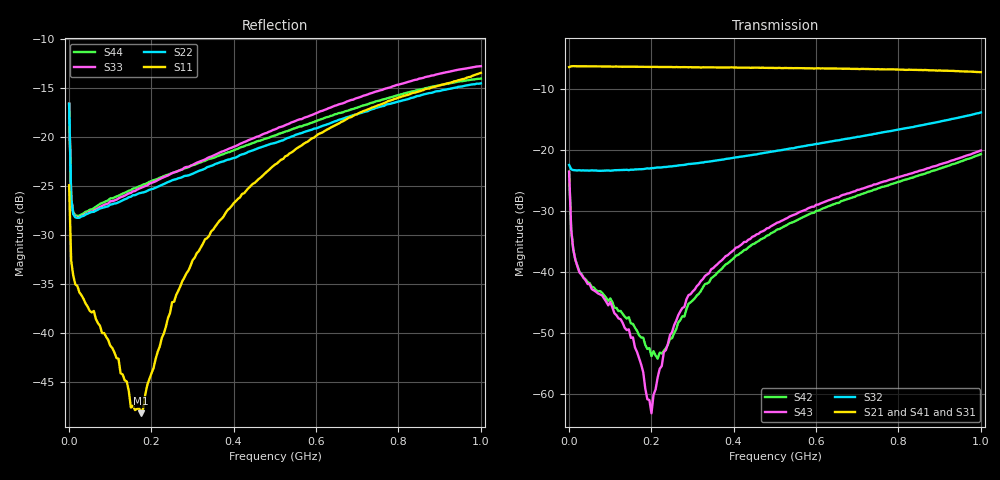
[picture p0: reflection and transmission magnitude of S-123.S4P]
!Agilent Technologies,E5071B,MY42300999,A.09.10
!Date: Thu Apr 13 17:00:39 2023
!Data & Calibration Information:
!Freq	S11:SOLT4(ON)	S12:SOLT4(ON)	S13:SOLT4(ON)	S14:SOLT4(ON)
!	S21:SOLT4(ON)	S22:SOLT4(ON)	S23:SOLT4(ON)	S24:SOLT4(ON)
!	S31:SOLT4(ON)	S32:SOLT4(ON)	S33:SOLT4(ON)	S34:SOLT4(ON)
!	S41:SOLT4(ON)	S42:SOLT4(ON)	S43:SOLT4(ON)	S44:SOLT4(ON)
# Hz S dB R 50
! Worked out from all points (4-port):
!   201 points, 1 MHz to 1 GHz, reference 50 ohm
!   strongest paths, dB at 1 MHz, 250.8 MHz, 500.5 MHz, 750.2 MHz, 1 GHz:
!     S21: -6.4, -6.4, -6.5, -6.7, -7.2
!     S41: -6.4, -6.4, -6.5, -6.8, -7.3
!     S31: -6.4, -6.4, -6.6, -6.9, -7.4
!     S32: -22.4, -22.6, -20.2, -17.2, -13.8
!     S43: -23.5, -49.8, -32.1, -25.5, -20.1
!     S42: -23.5, -50.8, -33.3, -26.3, -20.6
!   lowest |S11| = -48.2 dB at 175.8 MHz (marker M1), VSWR 1.01, Z = 50.3 + j0.268 ohm
!   |S11| at or under -10 dB: start of sweep to end of sweep
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1000000  -24.90 130.2  -6.41 2.4  -6.39 2.3  -6.41 2.4
         -6.39 2.3  -16.57 114.7  -22.42 -177.8  -23.51 -41.5
         -6.39 2.3  -22.42 -177.8  -16.54 114.7  -23.52 -41.7
         -6.40 2.4  -23.54 -41.4  -23.52 -41.6  -16.64 114.5
2.5975e7  -35.84 151.3  -6.26 -4.6  -6.27 -4.6  -6.25 -4.6
          -6.26 -4.6  -28.21 24.6  -23.30 174.2  -39.98 -39.8
          -6.25 -4.6  -23.29 174.0  -28.15 25.7  -40.01 -39.1
          -6.26 -4.6  -39.93 -40.3  -40.01 -38.8  -27.99 25.8
1.75825e8  -48.20 43.3  -6.35 -31.2  -6.37 -31.3  -6.32 -31.1
           -6.33 -31.1  -25.67 -9.5  -23.10 147.8  -50.66 -83.3
           -6.35 -31.3  -23.11 147.8  -25.15 -5.6  -55.18 -71.6
           -6.33 -31.1  -50.69 -85.0  -55.11 -73.3  -24.94 -2.2
2.008e8  -44.10 4.1  -6.36 -35.5  -6.39 -35.6  -6.34 -35.5
         -6.37 -35.5  -25.30 -12.9  -22.95 143.7  -53.83 -114.2
         -6.40 -35.9  -22.94 143.7  -24.66 -8.9  -63.06 -146.5
         -6.37 -35.6  -53.73 -116.9  -63.10 -148.8  -24.47 -5.3
2.9071e8  -33.59 -41.1  -6.42 -51.5  -6.48 -51.8  -6.41 -51.6
          -6.42 -51.5  -23.89 -25.6  -22.29 130.0  -45.21 146.3
          -6.44 -51.8  -22.27 130.0  -23.02 -20.9  -43.70 127.7
          -6.40 -51.6  -45.16 146.2  -43.73 128.2  -23.05 -17.2
4.2058e8  -25.79 -72.8  -6.49 -75.1  -6.55 -75.6  -6.47 -75.3
          -6.47 -75.1  -21.74 -44.4  -21.05 111.9  -36.71 112.3
          -6.54 -75.5  -21.04 111.9  -20.58 -39.3  -35.42 105.3
          -6.48 -75.3  -36.67 111.9  -35.38 104.9  -20.97 -35.2
1e9  -13.42 113.2  -7.23 157.2  -7.39 155.2  -7.30 155.2
     -7.22 157.3  -14.49 -122.8  -13.83 47.2  -20.64 30.2
     -7.42 155.0  -13.82 47.0  -12.73 -120.6  -20.04 33.5
     -7.29 155.3  -20.64 30.3  -20.05 33.6  -14.00 -119.4
